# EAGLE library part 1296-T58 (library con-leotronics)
1.27mm SINGLE ROW FEMALE SOCKET Source: http://www.leotronics.co.uk/Conexcon/Data%20Sheets/sec.%20A/1296ing.pdf
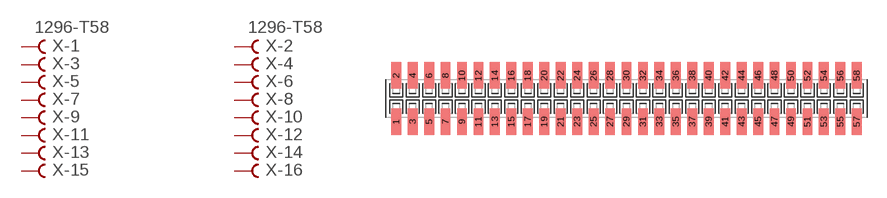
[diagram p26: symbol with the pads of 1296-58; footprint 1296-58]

Designator prefix X; gates -1=FVAL -2=FVAL -3=F -4=F -5=F -6=F -7=F -8=F -9=F -10=F -11=F -12=F -13=F -14=F -15=F -16=F -17=F -18=F -19=F -20=F -21=F -22=F -23=F -24=F -25=F -26=F -27=F -28=F -29=F -30=F -31=F -32=F -33=F -34=F -35=F -36=F -37=F -38=F -39=F -40=F -41=F -42=F -43=F -44=F -45=F -46=F -47=F -48=F -49=F -50=F -51=F -52=F -53=F -54=F -55=F -56=F -57=F -58=F

## 1296-T58 (OC_FARNELL: unknown; OC_NEWARK: unknown)  [1296-58]
1  -1:B  pas
2  -2:B  pas
3  -3:B  pas
4  -4:B  pas
5  -5:B  pas
6  -6:B  pas
7  -7:B  pas
8  -8:B  pas
9  -9:B  pas
10  -10:B  pas
11  -11:B  pas
12  -12:B  pas
13  -13:B  pas
14  -14:B  pas
15  -15:B  pas
16  -16:B  pas
17  -17:B  pas
18  -18:B  pas
19  -19:B  pas
20  -20:B  pas
21  -21:B  pas
22  -22:B  pas
23  -23:B  pas
24  -24:B  pas
25  -25:B  pas
26  -26:B  pas
27  -27:B  pas
28  -28:B  pas
29  -29:B  pas
30  -30:B  pas
31  -31:B  pas
32  -32:B  pas
33  -33:B  pas
34  -34:B  pas
35  -35:B  pas
36  -36:B  pas
37  -37:B  pas
38  -38:B  pas
39  -39:B  pas
40  -40:B  pas
41  -41:B  pas
42  -42:B  pas
43  -43:B  pas
44  -44:B  pas
45  -45:B  pas
46  -46:B  pas
47  -47:B  pas
48  -48:B  pas
49  -49:B  pas
50  -50:B  pas
51  -51:B  pas
52  -52:B  pas
53  -53:B  pas
54  -54:B  pas
55  -55:B  pas
56  -56:B  pas
57  -57:B  pas
58  -58:B  pas

## Footprint 1296-58 (pad centres in mm)
1.27mm SINGLE ROW FEMALE SOCKET Source: http://www.leotronics.co.uk/Conexcon/Data%20Sheets/sec.%20A/1296ing.pdf
smd 0.76 x 2.05: 1 -17.78,-1.78; 2 -17.78,1.78; 3 -16.51,-1.78; 4 -16.51,1.78; 5 -15.24,-1.78; 6 -15.24,1.78; 7 -13.97,-1.78; 8 -13.97,1.78; 9 -12.7,-1.78; 10 -12.7,1.78; 11 -11.43,-1.78; 12 -11.43,1.78; 13 -10.16,-1.78; 14 -10.16,1.78; 15 -8.89,-1.78; 16 -8.89,1.78; 17 -7.62,-1.78; 18 -7.62,1.78; 19 -6.35,-1.78; 20 -6.35,1.78; 21 -5.08,-1.78; 22 -5.08,1.78; 23 -3.81,-1.78; 24 -3.81,1.78; 25 -2.54,-1.78; 26 -2.54,1.78; 27 -1.27,-1.78; 28 -1.27,1.78; 29 0,-1.78; 30 0,1.78; 31 1.27,-1.78; 32 1.27,1.78; 33 2.54,-1.78; 34 2.54,1.78; 35 3.81,-1.78; 36 3.81,1.78; 37 5.08,-1.78; 38 5.08,1.78; 39 6.35,-1.78; 40 6.35,1.78; 41 7.62,-1.78; 42 7.62,1.78; 43 8.89,-1.78; 44 8.89,1.78; 45 10.16,-1.78; 46 10.16,1.78; 47 11.43,-1.78; 48 11.43,1.78; 49 12.7,-1.78; 50 12.7,1.78; 51 13.97,-1.78; 52 13.97,1.78; 53 15.24,-1.78; 54 15.24,1.78; 55 16.51,-1.78; 56 16.51,1.78; 57 17.78,-1.78; 58 17.78,1.78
